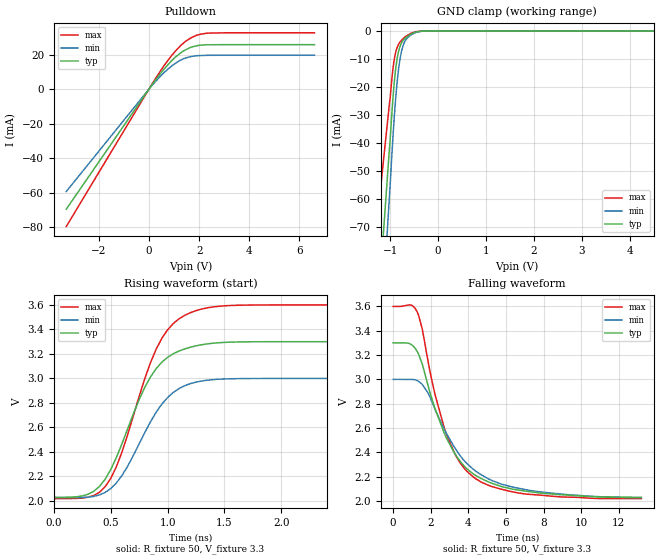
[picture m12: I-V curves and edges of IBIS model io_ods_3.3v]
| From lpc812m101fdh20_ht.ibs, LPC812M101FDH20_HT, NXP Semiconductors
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[Model]   io_ods_3.3v
Model_type I/O_open_drain
Vinl=9.900E-01
Vinh=2.310E+00
Vref=3.300E+00
Rref=1.000E+03
Cref=2.000E-11
Vmeas=1.650E+00
C_comp   8.440E-13   8.280E-13   8.600E-13
[Voltage Range]   3.300E+00   3.000E+00   3.600E+00
[POWER Clamp Reference]   3.300E+00   3.000E+00   3.600E+00
[GND Clamp Reference]   0.000E+00   0.000E+00   0.000E+00
[Pullup Reference]   3.300E+00   3.000E+00   3.600E+00
[Pulldown Reference]   0.000E+00   0.000E+00   0.000E+00
[Temperature Range]   25   105   -40
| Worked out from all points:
|   slope of the pulldown table from 0 to 0.495 V, typ, clamps not added: 51.2 ohm
|   GND clamp passes 1 mA (typ) near -0.56 V on its own axis
|   rising waveform, R_fixture 50, V_fixture 3.3: 20-80 % time 360ps typ, 355ps min, 352ps max; typ from 2.03 V to 3.3 V
|   falling waveform, R_fixture 50, V_fixture 3.3: 20-80 % time 2.11ns typ, 2.53ns min, 1.78ns max; typ from 3.3 V to 2.03 V
[GND Clamp]
-3.3V     -590.4mA   -705.8mA   -398.8mA
-1.02V    -42.46mA   -59.51mA   -26.24mA
-1V       -38.06mA   -54.12mA   -23.49mA
-960mV    -27.61mA   -42.2mA    -15.89mA
-920mV    -18.88mA   -31.48mA   -10.45mA
-880mV    -12.49mA   -22.47mA   -7.085mA
-820mV    -6.778mA   -12.65mA   -4.527mA
-780mV    -4.748mA   -8.414mA   -3.589mA
-720mV    -3.081mA   -4.622mA   -2.525mA
-560mV    -993.4uA   -1.291mA   -739uA
-280mV    0A         0A         0A
6.6V      0A         0A         0A
[Pulldown]
-3.3V     -69.61mA   -59.39mA   -79.67mA
160mV     3.297mA    2.77mA     3.818mA
560mV     10.84mA    8.974mA    12.7mA
900mV     16.39mA    13.31mA    19.41mA
1.16V     19.76mA    15.97mA    23.66mA
1.44V     22.62mA    17.89mA    27.44mA
1.66V     24.17mA    18.82mA    29.56mA
1.88V     25.03mA    19.33mA    31.09mA
2.4V      25.7mA     19.6mA     32.46mA
6.6V      25.77mA    19.62mA    32.62mA
[Rising Waveform]
R_fixture = 50
V_fixture = 3.3
V_fixture_min = 3
V_fixture_max = 3.6
0s        2.03V      2.028V     2.019V
300ps     2.055V     2.031V     2.031V
450ps     2.176V     2.069V     2.115V
600ps     2.47V      2.209V     2.402V
750ps     2.827V     2.466V     2.854V
850ps     3.013V     2.647V     3.13V
1ns       3.173V     2.844V     3.397V
1.15ns    3.241V     2.94V      3.515V
1.55ns    3.296V     2.997V     3.595V
3.55ns    3.3V       3V         3.6V
[Falling Waveform]
R_fixture = 50
V_fixture = 3.3
V_fixture_min = 3
V_fixture_max = 3.6
0s        3.3V       3V         3.6V
950ps     3.288V     3V         3.611V
1.3ns     3.224V     2.989V     3.548V
1.55ns    3.127V     2.959V     3.415V
2.2ns     2.774V     2.765V     2.896V
2.75ns    2.548V     2.581V     2.589V
3.45ns    2.351V     2.397V     2.342V
4.25ns    2.224V     2.262V     2.2V
7.4ns     2.074V     2.083V     2.053V
13.2ns    2.03V      2.028V     2.019V
[Ramp]
dV/dt_r   7.6204E-01/3.5770E-10   5.8333E-01/3.5330E-10   9.4867E-01/3.4960E-10
dV/dt_f   7.6204E-01/2.1066E-09   5.8333E-01/2.5229E-09   9.4867E-01/1.7695E-09
R_load = 50
